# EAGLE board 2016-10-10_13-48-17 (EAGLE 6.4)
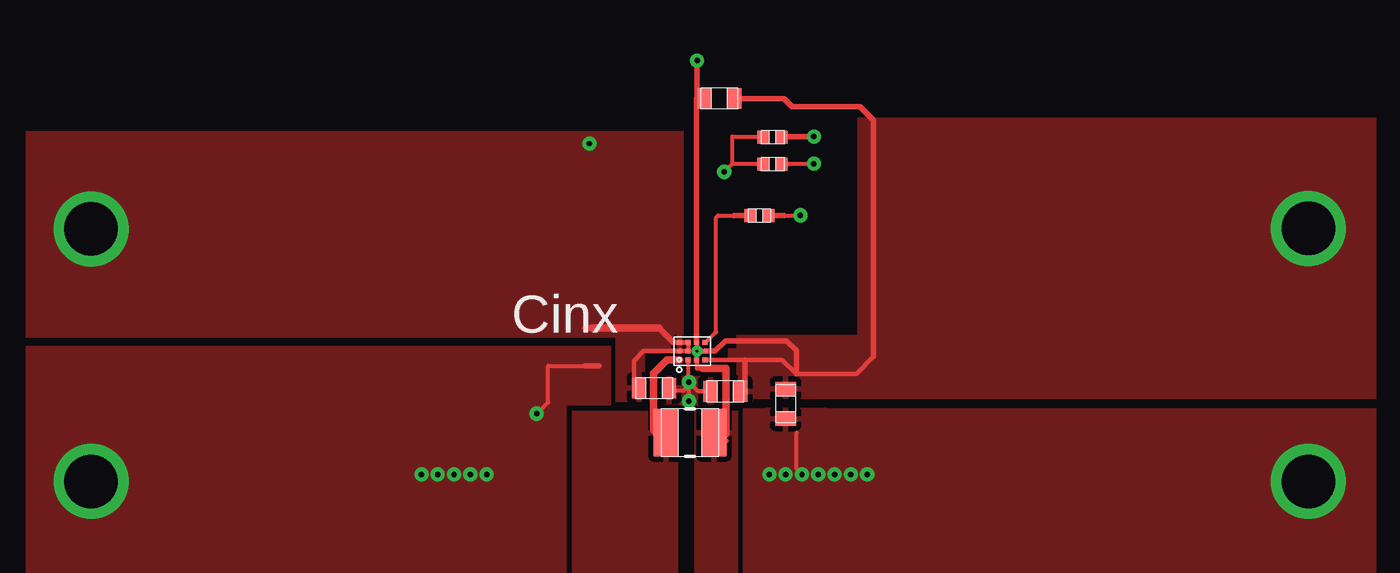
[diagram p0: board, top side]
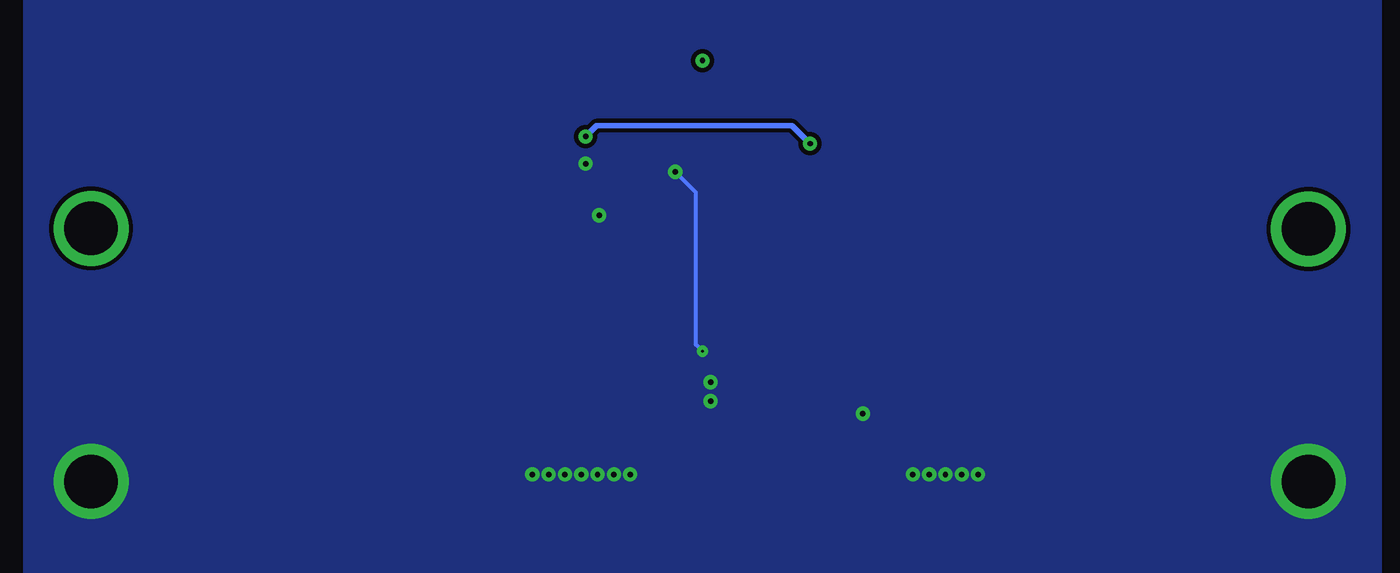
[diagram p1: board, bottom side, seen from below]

No outline drawn. Coordinates in mm, seen from the top.
Copper layers ((1*2)+(15*16)): TOP / INTERNAL1 / layer 15 / BOTTOM

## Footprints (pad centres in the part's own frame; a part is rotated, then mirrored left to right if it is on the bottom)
0603 = smd 0.66 x 0.965: 1 -0.699,0; 2 0.699,0
0402 = smd 0.559 x 0.61: 1 -0.419,0; 2 0.419,0
TP-1502 = drill 0.813 round: 1 0,0
1008 = smd 1.168 x 2.21: 1 -1.118,0; 2 1.118,0
YFF0012AFAF = smd 0.23 x 0.23: 1 -0.4,0.6; 2 0,0.6; 3 0.4,0.6; 4 -0.4,0.2; 5 0,0.2; 6 0.4,0.2; 7 -0.4,-0.2; 8 0,-0.2; 9 0.4,-0.2; 10 -0.4,-0.6; 11 0,-0.6; 12 0.4,-0.6

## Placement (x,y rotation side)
Cin  [0603]  55.78,41.96 0 top
Cout  [0603]  61.93,41.22 270 top
Coutx  [0603]  59.11,41.81 180 top
Css  [0402]  60.71,50.04 0 top
GND1  [TP-1502]  29.44,37.57 0 top
GND2  [TP-1502]  86.36,37.57 0 top
L1  [1008]  57.45,39.88 180 top
Rpfm  [0402]  61.32,52.43 0 top
Rpg  [0603]  58.83,55.5 180 top
Rpwm  [0402]  61.32,53.7 180 top
U1  [YFF0012AFAF]  57.56,43.69 90 top
VIN  [TP-1502]  29.44,49.38 0 top
VOUT  [TP-1502]  86.36,49.43 0 top

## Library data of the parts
Cin = ultra-librarian; RefDes: Cin; Type: LMK107BBJ106MAHT
Cout = ultra-librarian; RefDes: Cout; Type: CL10A106MQ8NNNC
Coutx = ultra-librarian; RefDes: Coutx; Type: CL10A106MQ8NNNC
Css = ultra-librarian; RefDes: Css; Type: GRM155R61A102KA01D
GND1 = ultra-librarian; RefDes: GND1; Type: TP-1502
GND2 = ultra-librarian; RefDes: GND2; Type: TP-1502
L1 = ultra-librarian; RefDes: L1; Type: LQM2HPN1R5MG0L
Rpfm = ultra-librarian; RefDes: Rpfm; Type: CRCW0402100KFKED
Rpg = ultra-librarian; RefDes: Rpg; Type: CRCW0603100KFKEA
Rpwm = ultra-librarian; RefDes: Rpwm; Type: CRCW0402100KFKED
U1 = ultra-librarian; RefDes: U1; Type: TPS63051YFFR
VIN = ultra-librarian; RefDes: VIN; Type: TP-1502
VOUT = ultra-librarian; RefDes: VOUT; Type: TP-1502

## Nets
0: Cin.2 Cout.2 Coutx.2 Css.2 GND1.1 GND2.1 Rpfm.1 Rpfm.2 Rpwm.2 U1.4 U1.8
2: Cin.1 Rpwm.1 U1.2 U1.3 U1.5 U1.6 VIN.1
3: Css.1 U1.12
4: Cout.1 Coutx.1 Rpg.1 U1.10 U1.11 VOUT.1
5: L1.1 U1.1
6: L1.2 U1.7
8: Rpg.2 U1.9

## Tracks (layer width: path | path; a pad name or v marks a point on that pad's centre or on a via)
0  (via drill 0.13 pad 0.23, 0.25 pad 0.56, 2.49 pad 3.48)
  TOP 0.198: 53.01,43 52.88,43 50.83,43 50.83,41.3 | v62.69,37.92 62.43,38.18 62.43,39.88 | 57.38,42.24 57.38,43.28 | 57.4,42.09 v57.4,42.24 57.81,41.83 58.24,41.83 | v57.4,41.35 57.4,42.09 | 56.62,41.86 57.17,41.86 57.4,42.09 | 61.85,52.45 v63.25,52.45 | 59.44,52.45 59.44,53.72 60.83,53.72 | v59.05,52.07 59.44,52.45 | 59.44,52.45 60.73,52.45 | 50.83,41.27 50.83,41.3 | v50.29,40.77 50.83,41.3 | 60.83,53.72 | 61.44,50.04 v62.61,50.04
  TOP 0.254: 52.55,43 53.21,43 | 61.01,50.02 61.85,50.02 | 60.71,53.71 60.94,53.71
  BOTTOM 0.198: v59.05,52.07 | v59.05,52.07 58.09,51.1 58.09,43.99 v57.78,43.69
  other vias: 61.16,37.92 61.93,37.92 63.45,37.92 64.21,37.92 65.74,37.92 64.97,37.92 44.91,37.92 45.67,37.92 46.43,37.92 47.19,37.92 47.96,37.92 86.36,37.59 29.46,37.59
  pour TOP (rank 5): 61.52,52.2 61.52,52.68 62.1,52.68 62.1,52.2
  pour TOP (rank 5): 60.53,52.2 60.53,52.68 61.11,52.68 61.11,52.2
  pour TOP (rank 5): 61.01,38.71 61.01,41.05 63.8,41.05 63.8,38.71
  pour TOP (rank 6): 57.48,43.28 57.48,43.28 57.48,43.31 57.45,43.33 57.45,43.33 57.43,43.36 57.43,43.36 57.4,43.38 57.38,43.38 57.38,43.38 57.35,43.38 57.33,43.38 57.3,43.36 57.3,43.36 57.28,43.33 57.28,43.33 57.25,43.31 57.25,43.28 57.25,43.28 57.25,43.26 57.25,43.23 57.28,43.21 57.28,43.21 57.3,43.18 57.3,43.18 57.33,43.15 57.35,43.15 57.38,43.15 57.38,43.15 57.4,43.15 57.43,43.18 57.43,43.18 57.45,43.21 57.45,43.21 57.48,43.23 57.48,43.26 57.48,43.28
  pour TOP (rank 6): 57.86,43.69 57.86,43.69 57.86,43.71 57.84,43.74 57.84,43.74 57.81,43.76 57.81,43.76 57.78,43.79 57.76,43.79 57.76,43.79 57.73,43.79 57.71,43.79 57.68,43.76 57.68,43.76 57.66,43.74 57.66,43.74 57.63,43.71 57.63,43.69 57.63,43.69 57.63,43.66 57.63,43.64 57.66,43.61 57.66,43.61 57.68,43.59 57.68,43.59 57.71,43.56 57.73,43.56 57.76,43.56 57.76,43.56 57.78,43.56 57.81,43.59 57.81,43.59 57.84,43.61 57.84,43.61 57.86,43.64 57.86,43.66 57.86,43.69
  pour TOP (rank 6): 56.24,42.52 58.65,42.52 58.6,41.15 56.24,41.15
  pour TOP (rank 6): 53.8,43.94 26.42,43.94 26.42,27.94 89.53,27.94 89.53,41.02 59.94,41.02 59.94,33.15 51.69,33.15 51.69,41.15 53.8,41.15
  pour BOTTOM: 26.04,26.16 89.53,26.16 89.53,61.59 26.04,61.59
2  (via drill 0.25 pad 0.56, 2.49 pad 3.48)
  TOP 0.203: 56.97,43.69 55.3,43.69 54.84,43.23 54.84,41.86 | 56.69,44.09 56.97,44.09 | 56.97,43.69 57.38,43.69 57.38,44.07 57.38,44.09 56.97,44.09 | 56.97,43.69 57,43.71 | 56.92,43.69 56.97,43.69 | 56.97,44.09 56.97,44.07 56.97,44.09
  TOP 0.254: 56.01,44.78 56.69,44.09 | 61.85,53.72 v63.25,53.72 | 52.55,44.78 53.21,44.78 | 61.7,53.71 61.92,53.71
  TOP 0.356: 52.88,44.78 56.01,44.78
  BOTTOM 0.254: 52.76,53.37 v52.76,53.39 53.59,54.23 62.74,54.23 v63.25,53.72
  other vias: 29.46,49.4
  pour TOP: 57.07,43.69 57.07,43.69 57.07,43.71 57.05,43.74 57.05,43.74 57.02,43.76 57.02,43.76 57,43.79 56.97,43.79 56.97,43.79 56.95,43.79 56.92,43.79 56.9,43.76 56.9,43.76 56.87,43.74 56.87,43.74 56.85,43.71 56.85,43.69 56.85,43.69 56.85,43.66 56.85,43.64 56.87,43.61 56.87,43.61 56.9,43.59 56.9,43.59 56.92,43.56 56.95,43.56 56.97,43.56 56.97,43.56 57,43.56 57.02,43.59 57.02,43.59 57.05,43.61 57.05,43.61 57.07,43.64 57.07,43.66 57.07,43.69
  pour TOP (rank 2): 57.48,43.69 57.48,43.69 57.48,43.71 57.45,43.74 57.45,43.74 57.43,43.76 57.43,43.76 57.4,43.79 57.38,43.79 57.38,43.79 57.35,43.79 57.33,43.79 57.3,43.76 57.3,43.76 57.28,43.74 57.28,43.74 57.25,43.71 57.25,43.69 57.25,43.69 57.25,43.66 57.25,43.64 57.28,43.61 57.28,43.61 57.3,43.59 57.3,43.59 57.33,43.56 57.35,43.56 57.38,43.56 57.38,43.56 57.4,43.56 57.43,43.59 57.43,43.59 57.45,43.61 57.45,43.61 57.48,43.64 57.48,43.66 57.48,43.69
  pour TOP (rank 2): 57.48,44.07 57.48,44.07 57.48,44.09 57.45,44.12 57.45,44.12 57.43,44.15 57.43,44.15 57.4,44.17 57.38,44.17 57.38,44.17 57.35,44.17 57.33,44.17 57.3,44.15 57.3,44.15 57.28,44.12 57.28,44.12 57.25,44.09 57.25,44.07 57.25,44.07 57.25,44.04 57.25,44.02 57.28,43.99 57.28,43.99 57.3,43.97 57.3,43.97 57.33,43.94 57.35,43.94 57.38,43.94 57.38,43.94 57.4,43.94 57.43,43.97 57.43,43.97 57.45,43.99 57.45,43.99 57.48,44.02 57.48,44.04 57.48,44.07
  pour TOP (rank 4): 53.98,44.32 53.98,41.33 55.35,41.33 55.35,43.59 57.18,43.59 57.18,44.32
  pour TOP (rank 4): 26.42,53.98 57.15,53.98 57.15,44.32 26.42,44.32
3
  TOP 0.198: 58.17,44.07 58.67,44.58 58.67,49.94 58.78,50.04 59.94,50.04 | 58.17,44.07
  TOP 0.254: 59.51,50.02 60.35,50.02
  pour TOP (rank 3): 58.27,44.07 58.27,44.07 58.27,44.09 58.24,44.12 58.24,44.12 58.22,44.15 58.22,44.15 58.19,44.17 58.17,44.17 58.17,44.17 58.14,44.17 58.12,44.17 58.09,44.15 58.09,44.15 58.06,44.12 58.06,44.12 58.04,44.09 58.04,44.07 58.04,44.07 58.04,44.04 58.04,44.02 58.06,43.99 58.06,43.99 58.09,43.97 58.09,43.97 58.12,43.94 58.14,43.94 58.17,43.94 58.17,43.94 58.19,43.94 58.22,43.97 58.22,43.97 58.24,43.99 58.24,43.99 58.27,44.02 58.27,44.04 58.27,44.07
4  (via drill 2.49 pad 3.48)
  TOP 0.203: 66.04,43.43 65.23,42.62 62.43,42.62 61.75,43.28 60.02,43.28 U1.10
  TOP 0.254: 60.02,41.83 60.02,43.28 | 59.84,55.5 61.85,55.5 62.23,55.12 65.41,55.12 66.04,54.48 66.04,43.43 | U1.11 58.62,43.69 59.11,44.17 61.98,44.17 62.43,43.71 62.43,42.62
  other vias: 86.36,49.43
  pour TOP: 58.27,43.28 58.27,43.28 58.27,43.31 58.24,43.33 58.24,43.33 58.22,43.36 58.22,43.36 58.19,43.38 58.17,43.38 58.17,43.38 58.14,43.38 58.12,43.38 58.09,43.36 58.09,43.36 58.06,43.33 58.06,43.33 58.04,43.31 58.04,43.28 58.04,43.28 58.04,43.26 58.04,43.23 58.06,43.21 58.06,43.21 58.09,43.18 58.09,43.18 58.12,43.15 58.14,43.15 58.17,43.15 58.17,43.15 58.19,43.15 58.22,43.18 58.22,43.18 58.24,43.21 58.24,43.21 58.27,43.23 58.27,43.26 58.27,43.28
  pour TOP (rank 2): 58.27,43.69 58.27,43.69 58.27,43.71 58.24,43.74 58.24,43.74 58.22,43.76 58.22,43.76 58.19,43.79 58.17,43.79 58.17,43.79 58.14,43.79 58.12,43.79 58.09,43.76 58.09,43.76 58.06,43.74 58.06,43.74 58.04,43.71 58.04,43.69 58.04,43.69 58.04,43.66 58.04,43.64 58.06,43.61 58.06,43.61 58.09,43.59 58.09,43.59 58.12,43.56 58.14,43.56 58.17,43.56 58.17,43.56 58.19,43.56 58.22,43.59 58.22,43.59 58.24,43.61 58.24,43.61 58.27,43.64 58.27,43.66 58.27,43.69
  pour TOP (rank 3): 59.64,41.33 59.64,42.34 60.4,42.34 60.4,41.33
  pour TOP (rank 4): 59.64,44.45 65.28,44.45 65.28,41.45 59.64,41.45
  pour TOP (rank 4): 65.28,41.45 65.28,54.61 89.53,54.61 89.53,41.45
  pour TOP (rank 5): 59.23,43.38 59.64,43.38 59.64,43.81 59.23,43.81
5
  TOP 0.203: 57.76,43.28 57.78,43.28 57.78,42.88 58.04,42.88
  TOP 0.254: 58.47,39.5 59.13,39.5
  TOP 0.356: 58.04,42.88 59.13,42.88 59.13,39.83 58.8,39.5
  pour TOP: 57.86,43.28 57.86,43.28 57.86,43.31 57.84,43.33 57.84,43.33 57.81,43.36 57.81,43.36 57.78,43.38 57.76,43.38 57.76,43.38 57.73,43.38 57.71,43.38 57.68,43.36 57.68,43.36 57.66,43.33 57.66,43.33 57.63,43.31 57.63,43.28 57.63,43.28 57.63,43.26 57.63,43.23 57.66,43.21 57.66,43.21 57.68,43.18 57.68,43.18 57.71,43.15 57.73,43.15 57.76,43.15 57.76,43.15 57.78,43.15 57.81,43.18 57.81,43.18 57.84,43.21 57.84,43.21 57.86,43.23 57.86,43.26 57.86,43.28
  pour TOP (rank 3): 59.69,40.89 59.69,33.32 57.66,33.32 57.66,40.89
6
  TOP 0.254: 55.93,39.5 56.59,39.5
  TOP 0.356: 56.26,39.5 55.75,40.01 55.75,42.65 56.39,43.28 56.97,43.28
  pour TOP: 57.07,43.28 57.07,43.28 57.07,43.31 57.05,43.33 57.05,43.33 57.02,43.36 57.02,43.36 57,43.38 56.97,43.38 56.97,43.38 56.95,43.38 56.92,43.38 56.9,43.36 56.9,43.36 56.87,43.33 56.87,43.33 56.85,43.31 56.85,43.28 56.85,43.28 56.85,43.26 56.85,43.23 56.87,43.21 56.87,43.21 56.9,43.18 56.9,43.18 56.92,43.15 56.95,43.15 56.97,43.15 56.97,43.15 57,43.15 57.02,43.18 57.02,43.18 57.05,43.21 57.05,43.21 57.07,43.23 57.07,43.26 57.07,43.28
  pour TOP (rank 3): 51.94,40.89 56.9,40.89 56.9,33.32 51.94,33.32
8  (via drill 0.25 pad 0.56)
  TOP 0.254: 57.76,44.07 57.76,55.5 57.78,55.52 v57.78,57.28
  pour TOP (rank 2): 57.86,44.07 57.86,44.07 57.86,44.09 57.84,44.12 57.84,44.12 57.81,44.15 57.81,44.15 57.78,44.17 57.76,44.17 57.76,44.17 57.73,44.17 57.71,44.17 57.68,44.15 57.68,44.15 57.66,44.12 57.66,44.12 57.63,44.09 57.63,44.07 57.63,44.07 57.63,44.04 57.63,44.02 57.66,43.99 57.66,43.99 57.68,43.97 57.68,43.97 57.71,43.94 57.73,43.94 57.76,43.94 57.76,43.94 57.78,43.94 57.81,43.97 57.81,43.97 57.84,43.99 57.84,43.99 57.86,44.02 57.86,44.04 57.86,44.07

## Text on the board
ASSYNOTES: Cinx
